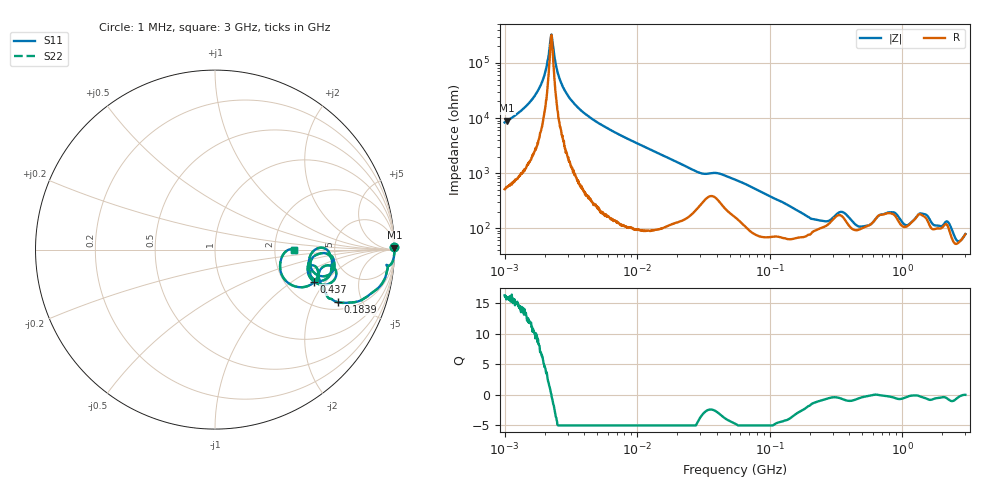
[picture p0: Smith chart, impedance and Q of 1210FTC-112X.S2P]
!s-Parameter Generated by FASTRON Sdn. Bhd.
!FASTRON P/N : 1210FTC-112X
!Keysight Technologies: E4991B_MY54100416_A.01.15
!Date created: Mon Dec 11 09:54:32 2023
!Version  : Rev00 Mon Dec 11 09:54:32 2023
!Data & Calibration Information:
!Freq	S11	S21	S12	S22
!PortZ  Port1:50+j0  Port2:50+j0
!When reading reference impedance value at option line is always used.
! Remarks : This data is being provided solely for informational purposes.
# Hz S dB R 50
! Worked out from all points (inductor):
!   1601 points, 1 MHz to 3 GHz, reference 50 ohm
!   read as one part in series: L = 1.06 mH near 1.041 MHz
!   highest Q = 16.1 at 1.046 MHz (marker M1), where L = 1.35 mH
!   self-resonance near 2.249 MHz
!   S11 on the Smith chart (normalised r, x): 1 MHz: open; 183.9 MHz: 2.40, -3.19; 437 MHz: 2.85, -1.54; 3 GHz: 2.56, -0.00
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1000000  -0.01 0.7  -38.40 -85.8  -38.40 -85.8  -0.01 0.7
1046065  -0.01 0.6  -38.99 -85.7  -38.99 -85.7  -0.01 0.6
1769069  -0.00 0.2  -49.66 -83.6  -49.66 -83.6  -0.00 0.2
1994811  -0.00 0.1  -55.43 -77.7  -55.43 -77.7  -0.00 0.1
2249358  -0.00 0.0  -70.16 -7.7  -70.16 -7.7  -0.00 0.0
2511129  -0.00 -0.1  -56.53 78.3  -56.53 78.3  -0.00 -0.1
2720446  -0.00 -0.1  -51.86 83.1  -51.86 83.1  -0.00 -0.1
3804036  -0.00 -0.4  -42.60 87.3  -42.60 87.3  -0.00 -0.4
1.447069e7  -0.02 -2.5  -27.19 85.1  -27.19 85.1  -0.02 -2.5
2.90111e7  -0.23 -5.3  -20.49 71.3  -20.49 71.3  -0.23 -5.3
5.477226e7  -0.30 -7.1  -17.92 70.8  -17.92 70.8  -0.30 -7.1
1.838549e8  -2.53 -23.2  -7.34 43.2  -7.34 43.2  -2.53 -23.2
2.083556e8  -3.48 -22.1  -6.84 33.6  -6.84 33.6  -3.48 -22.1
3.436571e8  -3.30 -10.0  -9.19 20.0  -9.19 20.0  -3.30 -10.0
4.369573e8  -4.72 -18.0  -6.34 21.8  -6.34 21.8  -4.72 -18.0
6.140682e8  -4.82 0.8  -7.42 -1.0  -7.42 -1.0  -4.82 0.8
7.925923e8  -3.56 -4.8  -9.28 9.3  -9.28 9.3  -3.56 -4.8
9.682285e8  -4.22 -14.0  -7.34 20.2  -7.34 20.2  -4.22 -14.0
1.268618e9  -4.34 -1.8  -8.08 2.8  -8.08 2.8  -4.34 -1.8
2.371269e9  -5.59 -23.5  -5.05 22.0  -5.05 22.0  -5.59 -23.5
2.660507e9  -8.59 -12.7  -3.85 7.3  -3.85 7.3  -8.59 -12.7
3e9  -7.18 -0.0  -5.00 0.0  -5.00 0.0  -7.18 -0.0
